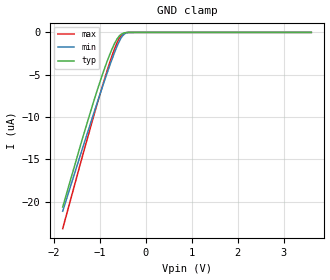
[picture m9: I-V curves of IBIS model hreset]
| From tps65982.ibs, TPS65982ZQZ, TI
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|   hreset Model
[Model]   hreset
Model_type   Input
Vinl = 0.63
Vinh = 1.25
|   typ   min   max
|   (nom PVT)   (fast PVT)   (slow PVT)
C_comp   2.476e-11   2.423e-11   2.599e-11
[Voltage Range]   1.8   1.7   1.9
[Temperature Range]   27   125   -40
[Power Clamp Reference]   1.8   1.7   1.9
[GND Clamp Reference]   0   0   0
[GND Clamp]
|   Voltage   I(typ)   I(min)   I(max)
-1.8V     -20.64uA   -21.12uA   -23.19uA
-1.348V   -12.11uA   -13.33uA   -14.16uA
-1.135V   -8.295uA   -9.723uA   -10.04uA
-914.4mV  -4.615uA   -6.07uA    -5.924uA
-785.1mV  -2.702uA   -4.02uA    -3.671uA
-673.3mV  -1.307uA   -2.36uA    -1.925uA
-578.3mV  -467.5nA   -1.134uA   -758.6nA
-496.1mV  -116.1nA   -380nA     -191.9nA
-407.3mV  -15.42nA   -58.02nA   -20.4nA
-180mV    0A         0A         0A
3.6V      0A         0A         0A
[POWER Clamp]
|   Voltage   I(typ)   I(min)   I(max)
-1.8V     0A         0A         0A
0V        0A         0A         0A
3.6V      0A         0A         0A
